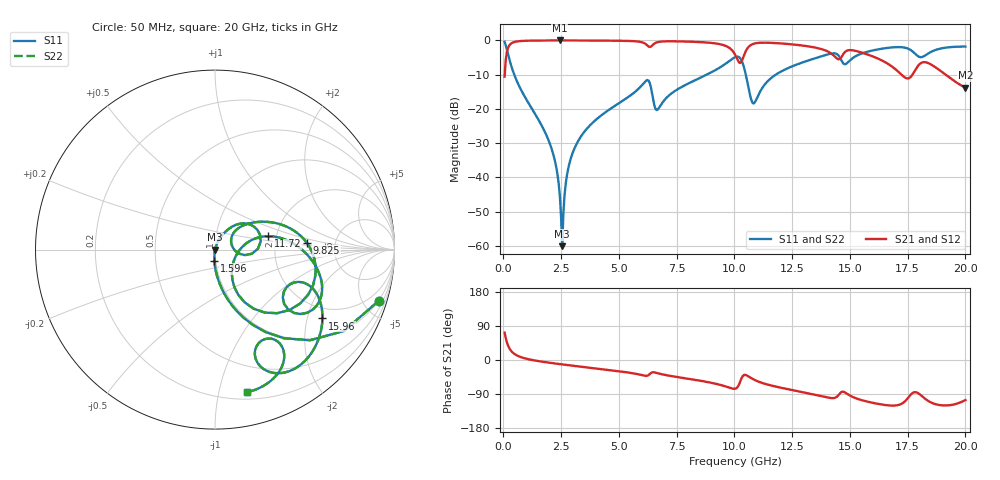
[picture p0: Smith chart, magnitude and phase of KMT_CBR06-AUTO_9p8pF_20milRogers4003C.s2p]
! Data measured by Modelithics Inc. support@modelithics.com 813-866-6335
! KEMET CBR06-AUTO 9.8pF, Pad Width= 0.851mm, Pad Length= 0.64mm, Pad Gap= 0.62mm, 20mil Rogers 4003C substrate Data, January 2022
# hz S ma R 50
! 2 Port Network Data from SP1.SP block
! freq  magS11  angS11  magS21  angS21  magS12  angS12  magS22  angS22
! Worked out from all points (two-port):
!   401 points, 50 MHz to 20 GHz, reference 50 ohm
!   highest |S21| = -0.01 dB at 2.444 GHz (marker M1); lowest = -13.8 dB at 20 GHz (marker M2)
!   |S21| within 3 dB of the highest: 163.6 MHz to 9.914 GHz (9.75 GHz wide, 194 % of centre); 10.5 GHz to 13.97 GHz (3.47 GHz wide, 28.4 % of centre)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
!   lowest |S11| = -60.0 dB at 2.544 GHz (marker M3), VSWR 1.00, Z = 50.1 - j0.00318 ohm
!   |S11| at or under -10 dB: 468.5 MHz to 8.796 GHz (8.327 GHz wide, 180 % of centre); 10.49 GHz to 11.79 GHz (1.294 GHz wide, 11.6 % of centre)
!   |S22| runs from -60.0 to -0.4 dB; largest |S21 - S12| = 0
!   S11 on the Smith chart (normalised r, x): 50 MHz: 0.98, -6.37; 1.596 GHz: 0.99, -0.12; 9.825 GHz: 3.07, +0.31; 11.72 GHz: 1.81, +0.30; 15.96 GHz: 1.60, -2.49; 20 GHz: 0.26, -1.22
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5e7  0.955 -17.5  0.2962 72.5  0.2962 72.5  0.955 -17.5
4.49e8  0.329 -72.7  0.9437 17.2  0.9437 17.2  0.329 -72.7
1.596125e9  0.0624 -93.0  0.9972 -3.7  0.9972 -3.7  0.0624 -93.0
2.194625e9  0.01948 -96.2  0.9988 -8.9  0.9988 -8.9  0.01948 -96.2
2.444e9  0.005276 -90.4  0.9989 -10.9  0.9989 -10.9  0.005276 -90.4
2.54375e9  0.0009953 -1.8  0.9989 -11.6  0.9989 -11.6  0.0009953 -1.8
2.843e9  0.01543 72.3  0.9987 -13.9  0.9987 -13.9  0.01543 72.3
3.391625e9  0.04137 70.5  0.9978 -17.8  0.9978 -17.8  0.04137 70.5
6.184625e9  0.2598 25.7  0.8712 -41.9  0.8712 -41.9  0.2598 25.7
6.73325e9  0.1036 30.1  0.953 -35.8  0.953 -35.8  0.1036 30.1
9.8255e9  0.5134 4.2  0.7576 -73.8  0.7576 -73.8  0.5134 4.2
1.0025e10  0.5691 -9.7  0.6236 -75.9  0.6236 -75.9  0.5691 -9.7
1.037412e10  0.4472 -51.7  0.5565 -41.3  0.5565 -41.3  0.4472 -51.7
1.0823e10  0.1202 -23.0  0.8919 -51.1  0.8919 -51.1  0.1202 -23.0
1.172075e10  0.3054 14.2  0.9172 -69.2  0.9172 -69.2  0.3054 14.2
1.336662e10  0.532 -5.1  0.8017 -90.1  0.8017 -90.1  0.532 -5.1
1.471325e10  0.4622 -35.2  0.631 -83.6  0.631 -83.6  0.4622 -35.2
1.596012e10  0.711 -32.7  0.5897 -112.6  0.5897 -112.6  0.711 -32.7
1.670825e10  0.7838 -45.8  0.442 -120.0  0.442 -120.0  0.7838 -45.8
1.78055e10  0.6486 -69.6  0.3591 -84.9  0.3591 -84.9  0.6486 -69.6
1.835412e10  0.6331 -55.4  0.4724 -106.6  0.4724 -106.6  0.6331 -55.4
2e10  0.8144 -77.3  0.2051 -105.8  0.2051 -105.8  0.8144 -77.3
